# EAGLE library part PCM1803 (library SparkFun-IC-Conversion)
PCM1803ADB STEREO ADC 24-bit Datasheet SparkFun Products none stock = 62
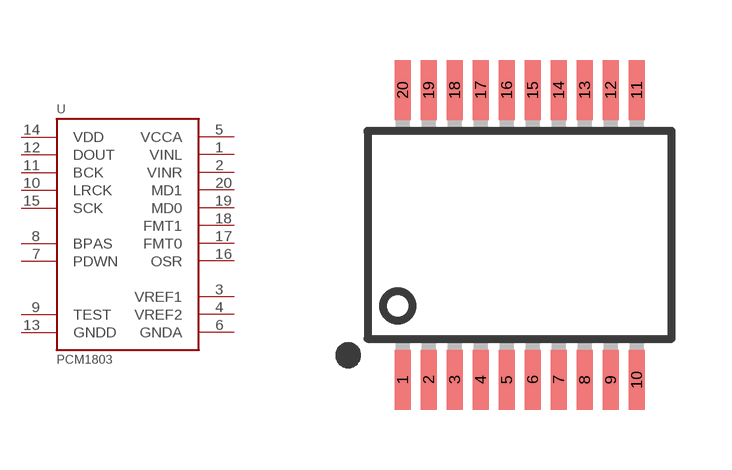
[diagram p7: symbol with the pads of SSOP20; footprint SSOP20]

Designator prefix U

## PCM1803SMD (PROD_ID: IC-09251; VALUE: PCM1803)  [SSOP20]
1  VINL
2  VINR
3  VREF1
4  VREF2
5  VCCA
6  GNDA
7  PDWN
8  BPAS
9  TEST
10  LRCK
11  BCK
12  DOUT
13  GNDD
14  VDD
15  SCK
16  OSR
17  FMT0
18  FMT1
19  MD0
20  MD1

## Footprint SSOP20 (pad centres in mm)
Shrink Small Outline Package package type SS
smd 0.4 x 1.5: 1 -2.925,-3.625; 2 -2.275,-3.625; 3 -1.625,-3.625; 4 -0.975,-3.625; 5 -0.325,-3.625; 6 0.325,-3.625; 7 0.975,-3.625; 8 1.625,-3.625; 9 2.275,-3.625; 10 2.925,-3.625; 11 2.925,3.625; 12 2.275,3.625; 13 1.625,3.625; 14 0.975,3.625; 15 0.325,3.625; 16 -0.325,3.625; 17 -0.975,3.625; 18 -1.625,3.625; 19 -2.275,3.625; 20 -2.925,3.625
